|   This file is an IBIS representation of the   |
|   CDCU877A provided by Texas Instruments   |
| This file contains preliminary package information for the following types:
|  uBGA 52-ball (GQL) package as [Component] cdcu877agql
|   MLF 40-pin  (RTB) package as [Component] cdcu877artb
|=================== Header Section -------------------------------------------|
[IBIS Ver]   3.2
[File Name]   cu877a_14.ibs
[File Rev]   2.3
[Date]   16 Apr 2004 | Last modified
|   20 Aug 2002 | Created
[Source]   This file originated at Texas Instruments
|   this file was generated based on simulation results of TI-Spice
|REVISON LOG:02 initial version
|   03 completely revised new model by Product Engineering
|   04 added package designator for bga, mlf package and combined them
|   to one model. Corrected CK/CK- to reflect passive pull-down.
|   05 added rising and falling waveforms.
|   06 new ouput buffers.
|   07 corrected ramp rates
|   08 CDCU877 PLL revised for A-DIE and C-DIE characteristics
|   Package parasitics added for BGA package.
|   09 Added per pin package paracitics for uBGA and MLF package,
|   changed componnent name to "RTB" for MLF-package,
|   corrected differential pin assignment.
|   Removed A-DIE references.
|   12 Correlated to real silicon with 2pF load und lossy option
|   enabled in linesim.
|   14 Corrected slew rate to latest CHAR-DATA
[Notes]
[Disclaimer]
(C) Copyright Texas Instruments Incorporated 2003
   All rights reserved
  Texas Instruments Incorporated hereby grants the user of this IBIS
model a non-exclusive, nontransferable license to use this IBIS model
under the following terms.  Before using this IBIS model, the user
should read this license.  If the user does not accept these terms,
the IBIS model should be returned to Texas Instruments within 30 days.
  The user is granted this license only to use the IBIS model and
is not granted rights to sell, load, rent, lease or license the IBIS
model in whole or in part, or in modified form to anyone other than
user.  User may modify the IBIS model to suit its specific applications
but rights to derivative works and such modifications shall belong to
Texas Instruments.
  This IBIS model is provided on an "AS IS" basis and Texas Instruments
makes absolutely no warranty with respect to the information contained
herein.  TEXAS INSTRUMENTS DISCLAIMS AND CUSTOMER WAIVES ALL WARRANTIES,
EXPRESS OR IMPLIED, INCLUDING WARRANTIES OF MERCHANTABILITY OR FITNESS
FOR A PARTICULAR PURPOSE. The entire risk as to quality and performance
is with the Customer. ACCORDINGLY, IN NO EVENT SHALL THE COMPANY BE LIABLE
FOR ANY DAMAGES, WHETHER IN CONTRACT OR TORT,INCLUDING ANY LOST PROFITS
OR OTHER INCIDENTAL, CONSEQUENTIAL, EXEMPLARY, OR PUNITIVE DAMAGES ARISING
OUT OF THE USE OR APPLICATION OF THE IBIS model provided in this package.
Further, Texas Instruments reserves the right to discontinue or make changes
without notice to any product herein to improve reliability, function, or
design. Texas Instruments does not convey any license under patent rights
or any other intellectual property rights, including those of third parties.
Contact Texas Instruments at ATTN: HPA-High Speed Communication & Control, HSCC
[Copyright]   Copyright (C)2003 Texas Instruments, All Rights Reserved
|------------------- End of Header Section ====================================|
|=================== Component Section ----------------------------------------|
| Component CDCU877AGQL, 52-ball, uBGA
[Component]   CDCU877AGQL   |Name of Device
[Manufacturer]  Texas Instruments
[Package]
|   typ   min   max
R_pkg   0.12Ohm   0.05Ohm   0.30Ohm
L_pkg   2.38nH   1.13nH   5.66nH
C_pkg   0.11pF   0.04pF   0.47pF
|pinout for uBGA package
[Pin] signal_name  model_name   R_pin   L_pin   C_pin
 D2   VDDQ   POWER   0.114Ohm   2.881nH   0.188pF
 C1   Y2-   Outbuf1   0.114Ohm   2.285nH   0.085pF
 D1   Y2   Outbuf1   0.094Ohm   1.872nH   0.079pF
 C2   GND   GND   0.080Ohm   2.098nH   0.257pF
 E1   CK   Inbuf_PD   0.087Ohm   1.754nH   0.074pF
 F1   CK-   Inbuf_PD   0.088Ohm   1.761nH   0.078pF
 F2   VDDQ   POWER   0.112Ohm   2.382nH   0.127pF
 G1   AGND   GND   0.051Ohm   1.129nH   0.079pF
 H1   AVDD   POWER   0.058Ohm   1.250nH   0.088pF
 G2   VDDQ   POWER   0.102Ohm   2.270nH   0.164pF
 H2   GND   GND   0.162Ohm   3.098nH   0.120pF
 J1   Y3   Outbuf1   0.134Ohm   2.519nH   0.052pF
 K1   Y3-   Outbuf1   0.134Ohm   2.519nH   0.052pF
 J2   GND   GND   0.122Ohm   2.311nH   0.053pF
 K2   Y4-   Outbuf1   0.124Ohm   2.347nH   0.060pF
 K3   Y4   Outbuf1   0.122Ohm   2.307nH   0.060pF
 G3   VDDQ   POWER   0.163Ohm   3.559nH   0.133pF
 K4   Y9   Outbuf1   0.123Ohm   2.322nH   0.060pF
 K5   Y9-   Outbuf1   0.126Ohm   2.381nH   0.060pF
 J5   GND   GND   0.071Ohm   1.447nH   0.220pF
 K6   Y8-   Outbuf1   0.140Ohm   2.627nH   0.051pF
 J6   Y8   Outbuf1   0.136Ohm   2.481nH   0.044pF
 G4   VDDQ   POWER   0.165Ohm   2.258nH   0.300pF
 D5   OS   Control   0.300Ohm   5.663nH   0.467pF
 F5   OE   Control   0.122Ohm   2.504nH   0.346pF
 H6   FBOUT   Outbuf1   0.110Ohm   2.156nH   0.104pF
 G6   FBOUT-   Outbuf1   0.100Ohm   1.961nH   0.074pF
 H5   GND   GND   0.153Ohm   3.024nH   0.173pF
 F6   FBIN-   Inbuf   0.089Ohm   1.779nH   0.075pF
 E6   FBIN   Inbuf   0.088Ohm   1.784nH   0.078pF
 E5   VDDQ   POWER   0.108Ohm   2.318nH   0.122pF
 D6   Y7   Outbuf1   0.095Ohm   1.887nH   0.079pF
 C6   Y7-   Outbuf1   0.106Ohm   2.129nH   0.083pF
 C5   GND   GND   0.088Ohm   1.872nH   0.139pF
 D4   VDDQ   POWER   0.134Ohm   3.050nH   0.200pF
 B6   Y6-   Outbuf1   0.134Ohm   2.524nH   0.053pF
 A6   Y6   Outbuf1   0.136Ohm   2.555nH   0.052pF
 B5   GND   GND   0.123Ohm   2.340nH   0.053pF
 A5   Y5   Outbuf1   0.125Ohm   2.367nH   0.060pF
 A4   Y5-   Outbuf1   0.123Ohm   2.322nH   0.061pF
 D3   VDDQ   POWER   0.159Ohm   3.476nH   0.128pF
 A3   Y0-   Outbuf1   0.122Ohm   2.306nH   0.061pF
 A2   Y0   Outbuf1   0.124Ohm   2.345nH   0.061pF
 B2   GND   GND   0.122Ohm   2.311nH   0.053pF
 A1   Y1   Outbuf1   0.131Ohm   2.474nH   0.052pF
 B1   Y1-   Outbuf1   0.129Ohm   2.444nH   0.052pF
[Diff_Pin]  inv_pin  vdiff   tdelay_typ  tdelay_min  tdelay_max
| The '+' pin is   Diff_pin,   the '-' pin is the   Inv_pin
| Receiver Pins  |  Receiver Vth = +/-300mV (DC, AC=0.6V)
E1   F1   0.3V   0ns   0ns   0ns   | CK  / CK-
E6   F6   0.3V   0ns   0ns   0ns   | FBIN/ FBIN-
| Driver Pins   |  Rload = xx ohm at xx termination
D1   C1   NA   0ns   0ns   0ns   | Y2 / Y2-
A1   B1   NA   0ns   0ns   0ns   | Y1 / Y1-
J1   K1   NA   0ns   0ns   0ns   | Y3 / Y3-
A2   A3   NA   0ns   0ns   0ns   | Y0 / Y0-
A5   A4   NA   0ns   0ns   0ns   | Y5 / Y5-
A6   B6   NA   0ns   0ns   0ns   | Y6 / Y6-
D6   C6   NA   0ns   0ns   0ns   | Y7 / Y7-
J6   K6   NA   0ns   0ns   0ns   | Y8 / Y8-
K4   K5   NA   0ns   0ns   0ns   | Y9 / Y9-
K3   K2   NA   0ns   0ns   0ns   | Y4 / Y4-
H6   G6   NA   0ns   0ns   0ns   | FBOUT / FBOUT-
[Model Selector]   Outbuf1
CDCU877C1_PLL C-DIE PLL_MODE (no buffer delay, no shift between splits in VT)
| Component CDCU877ARTB 40-pin MLF
[Component]   CDCU877ARTB   |Name of Device
[Manufacturer]  Texas Instruments
[Package]
|   typ   min   max
R_pkg   0.12Ohm   0.06Ohm   0.15Ohm
L_pkg   1.17nH   0.59nH   1.50nH
C_pkg   0.07pF   0.03pF   0.11pF
|pinning for MLF40 package
[Pin] signal_name  model_name   R_pin   L_pin   C_pin
  1   VDDQ   POWER   0.071Ohm   0.706nH   0.095pF
  2   Y2-   Outbuf2   0.133Ohm   1.319nH   0.080pF
  3   Y2   Outbuf2   0.124Ohm   1.229nH   0.111pF
  4   CK   Inbuf_PD   0.121Ohm   1.194nH   0.099pF
  5   CK-   Inbuf_PD   0.117Ohm   1.156nH   0.060pF
  6   VDDQ   POWER   0.117Ohm   1.157nH   0.070pF
  7   AGND   GND   0.060Ohm   0.592nH   0.071pF
  8   AVDD   POWER   0.062Ohm   0.609nH   0.072pF
  9   VDDQ   POWER   0.064Ohm   0.632nH   0.074pF
 10   GND   GND   0.143Ohm   1.419nH   0.078pF
 11   Y3   Outbuf2   0.146Ohm   1.442nH   0.071pF
 12   Y3-   Outbuf2   0.133Ohm   1.321nH   0.048pF
 13   Y4-   Outbuf2   0.128Ohm   1.267nH   0.085pF
 14   Y4   Outbuf2   0.121Ohm   1.195nH   0.063pF
 15   VDDQ   POWER   0.117Ohm   1.157nH   0.056pF
 16   Y9   Outbuf2   0.117Ohm   1.156nH   0.055pF
 17   Y9-   Outbuf2   0.121Ohm   1.195nH   0.056pF
 18   Y8-   Outbuf2   0.125Ohm   1.233nH   0.057pF
 19   Y8   Outbuf2   0.134Ohm   1.325nH   0.054pF
 20   VDDQ   POWER   0.071Ohm   0.700nH   0.076pF
 21   OS   Control   0.145Ohm   1.439nH   0.077pF
 22   OE   Control   0.133Ohm   1.318nH   0.084pF
 23   VDDQ   POWER   0.124Ohm   1.229nH   0.073pF
 24   FBOUT   Outbuf2   0.118Ohm   1.173nH   0.061pF
 25   FBOUT-   Outbuf2   0.116Ohm   1.152nH   0.073pF
 26   FBIN-   Inbuf   0.117Ohm   1.157nH   0.070pF
 27   FBIN   Inbuf   0.121Ohm   1.196nH   0.074pF
 28   VDDQ   POWER   0.128Ohm   1.272nH   0.075pF
 29   Y7   Outbuf2   0.139Ohm   1.375nH   0.081pF
 30   Y7-   Outbuf2   0.151Ohm   1.500nH   0.041pF
 31   VDDQ   POWER   0.071Ohm   0.705nH   0.081pF
 32   Y6-   Outbuf2   0.133Ohm   1.316nH   0.097pF
 33   Y6   Outbuf2   0.124Ohm   1.227nH   0.060pF
 34   Y5   Outbuf2   0.120Ohm   1.192nH   0.049pF
 35   Y5-   Outbuf2   0.117Ohm   1.156nH   0.054pF
 36   VDDQ   POWER   0.117Ohm   1.158nH   0.049pF
 37   Y0-   Outbuf2   0.121Ohm   1.198nH   0.033pF
 38   Y0   Outbuf2   0.129Ohm   1.274nH   0.025pF
 39   Y1   Outbuf2   0.134Ohm   1.330nH   0.101pF
 40   Y1-   Outbuf2   0.146Ohm   1.447nH   0.084pF
Pad   GND   GND   0.007Ohm   0.064nH   0.355pF
[Diff_Pin]  inv_pin  vdiff   tdelay_typ  tdelay_min  tdelay_max
| The '+' pin is   Diff_pin,   the '-' pin is the   Inv_pin
| Receiver Pins  |  Receiver Vth = +/-300mV (DC, AC=0.6V)
4   5   0.3V   0ns   0ns   0ns   | CK  / CK-
27   26   0.3V   0ns   0ns   0ns   | FBIN/ FBIN-
| Driver Pins   |  Rload = xx ohm at xx termination
3   2   NA   0ns   0ns   0ns   | Y2 / Y2-
11   12   NA   0ns   0ns   0ns   | Y3 / Y3-
14   13   NA   0ns   0ns   0ns   | Y4 / Y4-
16   17   NA   0ns   0ns   0ns   | Y9 / Y9-
19   18   NA   0ns   0ns   0ns   | Y8 / Y8-
24   25   NA   0ns   0ns   0ns   | FBOUT / FBOUT-
29   30   NA   0ns   0ns   0ns   | Y7 / Y7-
33   32   NA   0ns   0ns   0ns   | Y6 / Y6-
34   35   NA   0ns   0ns   0ns   | Y5 / Y5-
38   37   NA   0ns   0ns   0ns   | Y0 / Y0-
39   40   NA   0ns   0ns   0ns   | Y1 / Y1-
|------------------- End of Component Section ==============================
[Model Selector]   Outbuf2
CDCU877C1_PLL C-DIE PLL_MODE (no buffer delay, no shift between splits in VT)
| Models and submodels in the file (4): Inbuf (Input), Inbuf_PD (Input), Control (Input), CDCU877C1_PLL (Output)
